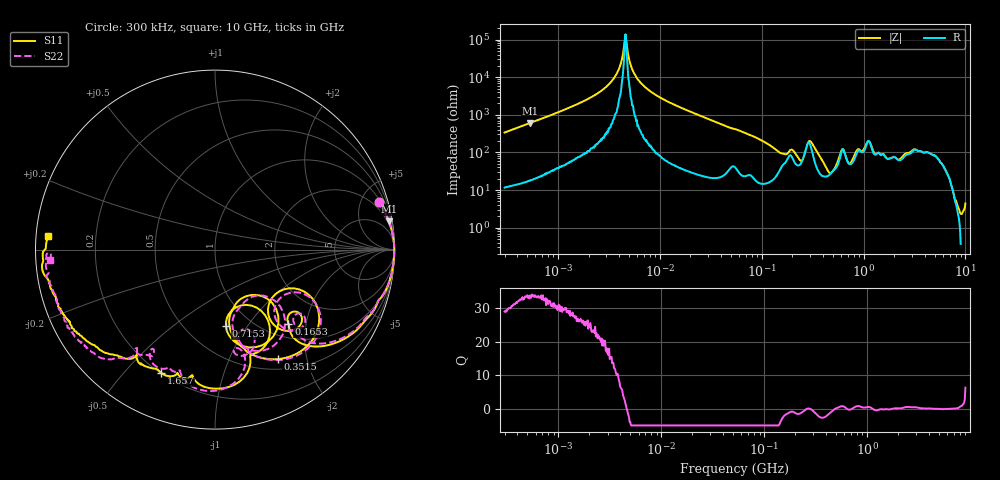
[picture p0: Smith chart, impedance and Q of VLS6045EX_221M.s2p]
! S-Parameter Data Generated by TDK Corporation
! Copyright(C) 2019 TDK Corporation.
! All Rights Reserved.
! TDK P/N: VLS6045EX-221M (Inductor)
! Property: L=220uH at 100kHz
! Size(LxWxT): 6x6x4.5mm
! Model Type: s2p (Touchstone File Format Version 1.0)
! Frequency: DC=Yes Start=0.3MHz Stop=10000MHz 802points Log-sweep
! Model Generated on May 10, 2019
! Port Assignments:
!  1 ---@@@--- 2
! Applicable Conditions:
!  Temperature = 25 degC
!  DC Bias Current = 0 A
!  Small Signal Operation
! Terms and conditions regarding TDK Simulation Models
! (1)This simulation model is being provided solely for informational purposes. Please refer to the specifications of the products in terms of detailed characteristics of such products.
! (2)In no event shall TDK Corporation of any of its subsidiaries be liable for any loss or damage arising, directly or indirectly,
!  From any information contained in this simulation model, including, but not limited to loss or damages arising from any inaccuracies, omissions or errors in connection with such information.
! (3)Any and all copyrights on this simulation model are owned by TDK Corporation.
!  Duplication or redistribution of this simulation model without prior written permission from TDK Corporation is prohibited.
! (4)This simulation model is subject to any modification or change without any prior notice.
! (5)Neither TDK Corporation nor any of its subsidiaries shall make any warranty, express or implied,
!  Including but not limited to the correctness, implied warranties of merchantability and fitness for a particular purpose with respect to this simulation models.
! (6)The use of this simulation model shall be deemed to have consented to the terms and conditions hereof.
# Hz S MA R 50
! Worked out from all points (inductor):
!   801 points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, 300 kHz to 10 GHz, reference 50 ohm
!   read as one part in series: L = 178 uH near 318.3 kHz
!   highest Q = 33.6 at 536 kHz (marker M1), where L = 180 uH
!   self-resonance near 4.549 MHz
!   S11 on the Smith chart (normalised r, x): 300 kHz: 1.28, +6.83; 165.3 MHz: 1.27, -1.59; 351.5 MHz: 0.64, -1.53; 715.3 MHz: 0.77, -0.80; 1.657 GHz: 0.20, -0.64; 10 GHz: 0.04, +0.04
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300000  0.9494 16.1  0.2809 -71.9  0.2809 -71.9  0.9493 16.1
535999  0.9814 9.2  0.1618 -79.1  0.1619 -79.1  0.9814 9.2
1713600  0.9972 2.5  0.04586 -85.4  0.04584 -85.4  0.9972 2.5
3464350  0.999 0.3  0.01168 -84.9  0.01159 -85.4  0.999 0.4
4611084  0.9992 -0.4  0.0007336 2.9  0.0007127 -0.5  0.9993 -0.4
5698586  0.9992 -1.0  0.008594 84.6  0.008601 84.6  0.9994 -1.0
9671944  0.9984 -2.8  0.03255 85.6  0.03255 85.7  0.9986 -2.7
5.477226e7  0.9521 -17.9  0.2253 66.8  0.2253 66.8  0.9538 -17.5
1.210198e8  0.8162 -41.0  0.4985 44.1  0.4985 44.1  0.8195 -39.3
1.653189e8  0.5825 -45.3  0.5692 17.3  0.5692 17.3  0.605 -43.1
2.663116e8  0.4929 -26.0  0.4918 -18.5  0.4918 -18.5  0.5266 -27.0
3.126428e8  0.7422 -44.2  0.3689 12.4  0.3689 12.4  0.7551 -44.6
3.514851e8  0.7028 -60.3  0.5294 13.0  0.5293 13.0  0.7115 -59.8
4.508285e8  0.4417 -79.3  0.7169 -13.2  0.7168 -13.2  0.4505 -77.3
5.497689e8  0.3255 -51.0  0.6596 -41.4  0.6596 -41.4  0.3352 -51.4
7.152593e8  0.4307 -81.9  0.5678 -38.7  0.5676 -38.7  0.524 -75.2
8.872678e8  0.5898 -60.2  0.3734 -68.4  0.373 -68.4  0.6117 -74.1
1.165098e9  0.7751 -88.3  0.2218 -57.9  0.2214 -57.9  0.7887 -91.8
1.657186e9  0.75 -113.4  0.2849 -72.1  0.2841 -71.9  0.7188 -119.4
1.767019e9  0.7415 -116.4  0.2896 -80.7  0.2887 -80.5  0.6764 -122.5
5.157474e9  0.9198 -158.1  0.0558 -128.2  0.05616 -128.7  0.9242 -152.7
1e10  0.9317 175.2  0.05288 -146.7  0.05263 -146.7  0.9201 -176.3
